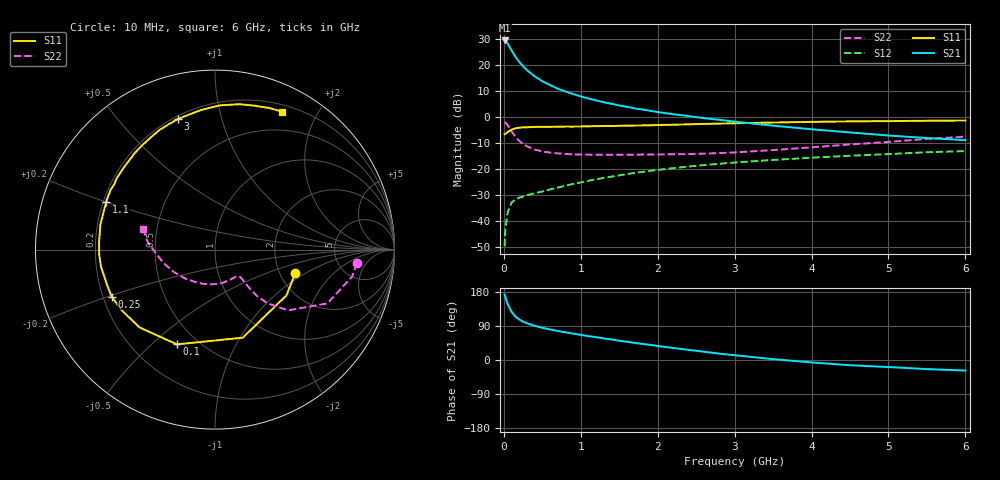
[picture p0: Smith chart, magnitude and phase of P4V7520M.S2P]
! SIEMENS Small Signal Semiconductors
! BFP182
! Si NPN RF Bipolar Junction Transistor in SOT143
! VCE = 0.75 V  IC = 20 mA
! Common Emitter S-Parameters:  March  1996
# GHz  S  MA  R  50
!  f  S11  S21  S12  S22
! GHz  MAG  ANG  MAG  ANG  MAG  ANG  MAG  ANG
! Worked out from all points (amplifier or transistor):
!   36 points, 10 MHz to 6 GHz, reference 50 ohm
!   highest |S21| = 29.4 dB at 10 MHz (marker M1)
!   |S21| within 3 dB of that: start of sweep to 84.69 MHz
!   unconditionally stable (mu >= 1): start of sweep to 15.25 MHz; 274.4 MHz to end of sweep
!   at 250 MHz: K = 0.93, MSG = 25.0 dB, |S12| = -30.6 dB
!   at 1.4 GHz: K = 2.03, MAG = 8.2 dB, |S12| = -22.9 dB
!   at 6 GHz: K = 1.58, MAG = -2.4 dB, |S12| = -13.1 dB
!   S11 on the Smith chart (normalised r, x): 10 MHz: 2.42, -0.82; 100 MHz: 0.39, -0.60; 250 MHz: 0.24, -0.21; 1.1 GHz: 0.21, +0.20; 3 GHz: 0.22, +0.73; 6 GHz: 0.28, +1.57
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0.01  0.4663 -16.5  29.43 173.1  0.0033 77.8  0.7943 -5.5
0.02  0.4729 -32.6  29.11 166.4  0.007 74.4  0.7785 -11.2
0.05  0.5145 -72.5  25.68 147.9  0.0147 62.5  0.6938 -25.6
0.1  0.5691 -111.9  19 127.4  0.0226 46.2  0.5299 -39.7
0.15  0.6038 -134.1  14.43 114.9  0.0261 40.8  0.4176 -45.7
0.2  0.6203 -147.0  11.44 107.0  0.0282 38.2  0.3471 -47.9
0.25  0.6325 -155.5  9.403 101.3  0.0296 37.6  0.3037 -48.3
0.3  0.633 -162.2  7.94 97.0  0.0314 38.3  0.2736 -48.1
0.4  0.6425 -171.5  6.052 90.2  0.0342 40.2  0.2364 -47.6
0.5  0.6461 -178.0  4.871 85.1  0.037 41.6  0.2172 -47.3
0.6  0.6474 176.4  4.107 80.7  0.0405 44.0  0.2072 -47.4
0.7  0.6487 171.6  3.497 76.7  0.044 45.9  0.1997 -48.4
0.9  0.6533 163.9  2.753 69.8  0.0517 48.3  0.1911 -51.5
1.1  0.6612 156.4  2.262 63.0  0.0595 49.5  0.1888 -55.7
1.5  0.6767 144.2  1.663 50.8  0.0757 49.0  0.1885 -65.7
1.7  0.6836 137.8  1.464 45.1  0.0842 48.8  0.1875 -71.7
2.2  0.7089 124.9  1.129 31.8  0.1037 45.5  0.1923 -88.1
3  0.7565 105.8  0.813 12.6  0.1333 38.1  0.2085 -117.5
3.5  0.7809 96.0  0.68 2.3  0.1494 33.2  0.2312 -135.6
4.5  0.8216 80.4  0.504 -13.8  0.1796 23.5  0.2962 -165.4
5.5  0.8452 68.9  0.394 -24.0  0.2102 14.1  0.3786 173.3
6  0.8548 63.9  0.359 -27.8  0.2208 8.6  0.4168 164.1
